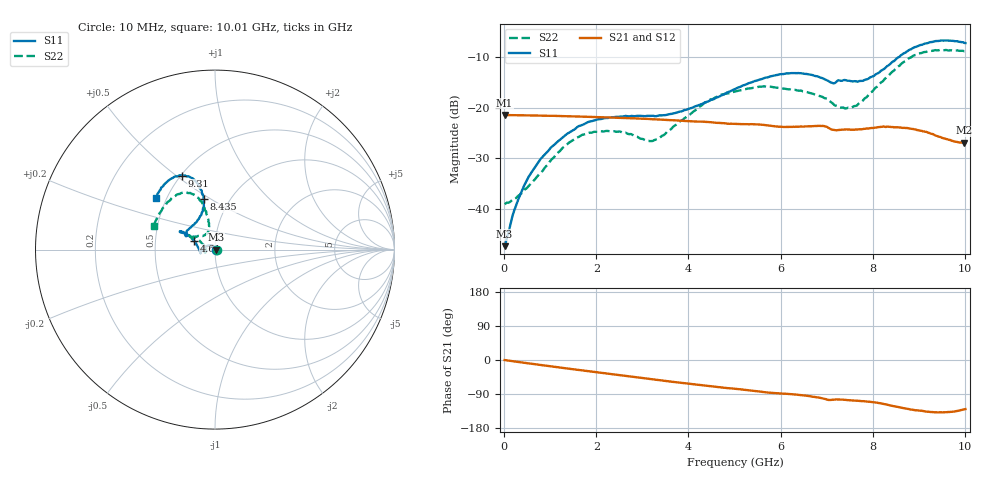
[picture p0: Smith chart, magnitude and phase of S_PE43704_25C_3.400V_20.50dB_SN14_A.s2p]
! Device ID: PE43704
! Dir: z:\PE43704\PE43704_Char_1_20130516\PE43704\AMB\3p400V\20p50dB
! Serial: 14
! Insertion: A
! Impedance: 50 ohm
! Temp: Amb
! VDD: 3.400V
! Attenuation Step: 20.50dB
! IDD: 1.139804e-01mA
#  Hz  S  RI  R  50
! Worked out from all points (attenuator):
!   401 points, 10 MHz to 10.01 GHz, reference 50 ohm
!   highest |S21| = -21.44 dB at 10 MHz (marker M1); lowest = -26.9 dB at 9.985 GHz (marker M2)
!   lowest |S11| = -47.4 dB at 10 MHz (marker M3), VSWR 1.01, Z = 50.4 + j0.0382 ohm
!   |S11| at or under -10 dB: start of sweep to 8.553 GHz
!   |S22| runs from -39.1 to -8.5 dB; largest |S21 - S12| = 0.00098
!   S11 on the Smith chart (normalised r, x): 10 MHz: 1.01, +0.00; 4.61 GHz: 0.79, +0.08; 8.435 GHz: 0.76, +0.46; 9.31 GHz: 0.51, +0.52; 10.01 GHz: 0.44, +0.31
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1e7  0.00423 0.000379  0.0847 -0.000249  0.0848 -0.000311  0.0111 0.000357
2.85e8  0.00129 0.0115  0.084 -0.00709  0.0841 -0.00709  0.00802 0.0104
5.85e8  -0.00901 0.0207  0.0827 -0.0143  0.0827 -0.0142  -0.00186 0.0177
1.035e9  -0.0338 0.0234  0.0796 -0.0244  0.0796 -0.0242  -0.0254 0.0178
1.36e9  -0.0523 0.0169  0.0763 -0.0312  0.0763 -0.0312  -0.0421 0.00995
1.685e9  -0.067 0.00592  0.0725 -0.0377  0.0726 -0.0377  -0.0536 -0.00159
2.26e9  -0.0783 -0.013  0.0645 -0.0477  0.0645 -0.0475  -0.0566 -0.0157
3.135e9  -0.0813 -0.0175  0.0499 -0.0592  0.0498 -0.0593  -0.047 -0.00142
3.36e9  -0.0832 -0.0117  0.0455 -0.0613  0.0457 -0.0612  -0.0491 0.00774
4.61e9  -0.1168 0.0484  0.0228 -0.0673  0.0229 -0.0673  -0.108 0.0689
5.01e9  -0.1363 0.0698  0.0168 -0.0671  0.0168 -0.0672  -0.1265 0.0708
5.96e9  -0.1878 0.1015  0.00242 -0.0648  0.00235 -0.0648  -0.1406 0.0697
6.685e9  -0.1887 0.0952  -0.00751 -0.0653  -0.00739 -0.0652  -0.1216 0.066
7.135e9  -0.1564 0.0791  -0.0155 -0.0584  -0.0155 -0.0583  -0.0805 0.0749
7.535e9  -0.1355 0.123  -0.0174 -0.0581  -0.0173 -0.0582  -0.0451 0.0888
7.86e9  -0.0959 0.1655  -0.0207 -0.0587  -0.0204 -0.0586  -0.0335 0.1219
8.36e9  -0.0621 0.2601  -0.0316 -0.0565  -0.0314 -0.0566  -0.0487 0.2068
8.435e9  -0.063 0.2799  -0.0333 -0.0552  -0.0333 -0.0551  -0.057 0.2225
8.86e9  -0.1026 0.3746  -0.0407 -0.0464  -0.0402 -0.0467  -0.1128 0.3037
9.31e9  -0.1834 0.4121  -0.0404 -0.0368  -0.0407 -0.0366  -0.2003 0.3098
9.985e9  -0.3231 0.2982  -0.0292 -0.0343  -0.0295 -0.0341  -0.3361 0.138
1.001e10  -0.3285 0.2901  -0.0288 -0.0348  -0.0293 -0.0349  -0.3404 0.1295
